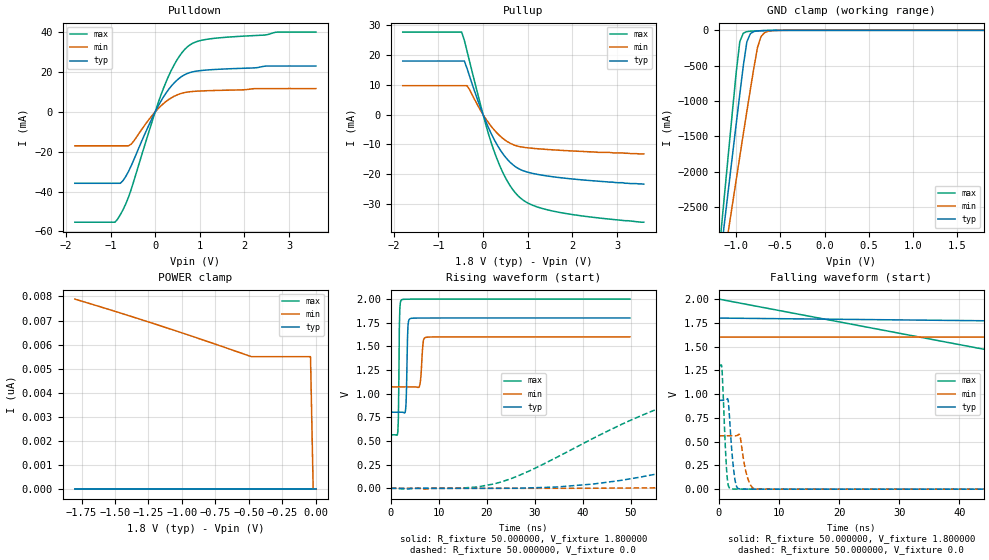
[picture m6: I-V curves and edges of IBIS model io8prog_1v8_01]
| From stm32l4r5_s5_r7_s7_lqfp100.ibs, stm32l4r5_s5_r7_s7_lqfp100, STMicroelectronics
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|   Model io8prog_1v8_01
[Model]  io8prog_1v8_01
Model_type I/O
Polarity   Non-Inverting
Enable   Active-Low
Vinl =   0.540000V
Vinh =   1.260000V
Vmeas =  0.900000V
Cref =   100.000000nF
Rref =   1.000000k
Vref =   1.800000V
C_comp   2.197300pF   2.162700pF   2.264100pF
[Temperature Range]   25.000000   0.125000k   -40.000000
[Pullup Reference]   1.800000V   1.600000V   2.000000V
[Pulldown Reference]   0.0V   0.0V   0.0V
[POWER Clamp Reference]   1.800000V   1.600000V   2.000000V
[GND Clamp Reference]   0.0V   0.0V   0.0V
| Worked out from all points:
|   slope of the pulldown table from 0 to 0.27 V, typ, clamps not added: 26.2 ohm
|   slope of the pullup table from 0 to 0.27 V, typ, clamps not added: 30.1 ohm
|   GND clamp passes 1 mA (typ) near -0.58 V on its own axis
|   rising waveform, R_fixture 50.000000, V_fixture 1.800000: 20-80 % time 248ps typ, 394ps min, 184ps max; typ from 0.804 V to 1.8 V
|   rising waveform, R_fixture 50.000000, V_fixture 0.0: 20-80 % time 65.2ns typ, 116ns min, 36.2ns max; typ from 0 V to 0.934 V
|   falling waveform, R_fixture 50.000000, V_fixture 1.800000: 20-80 % time 75.8ns typ, 121ns min, 63.2ns max; typ from 1.8 V to 0.804 V
|   falling waveform, R_fixture 50.000000, V_fixture 0.0: 20-80 % time 711ps typ, 1.02ns min, 545ps max; typ from 0.934 V to 0 V
[Pulldown]
|Voltage   I(typ)   I(min)   I(max)
-1.8V     -35.82mA   -17.03mA   -55.34mA
-900mV    -35.82mA   -17.03mA   -55.34mA
-840mV    -35.82mA   -17.03mA   -53.76mA
-720mV    -34.49mA   -17.03mA   -49.08mA
-540mV    -27.18mA   -16.22mA   -39.07mA
-60mV     -2.756mA   -1.584mA   -4.227mA
240mV     9.353mA    5.171mA    14.85mA
480mV     15.75mA    8.427mA    25.77mA
720mV     19.29mA    9.947mA    32.62mA
960mV     20.57mA    10.43mA    35.5mA
1.32V     21.27mA    10.74mA    36.91mA
3.6V      23.03mA    11.73mA    40.05mA
[Pullup]
|Voltage   I(typ)   I(min)   I(max)
-1.8V     18.05mA    9.741mA    27.78mA
-480mV    18.05mA    9.741mA    27.78mA
-420mV    18.05mA    9.741mA    25.03mA
-360mV    15.57mA    9.741mA    21.38mA
60mV      -2.268mA   -1.401mA   -3.341mA
240mV     -8.143mA   -5.004mA   -12mA
360mV     -11.31mA   -6.914mA   -16.72mA
540mV     -15mA      -9.056mA   -22.31mA
840mV     -18.52mA   -10.83mA   -28.11mA
1.14V     -19.87mA   -11.38mA   -30.67mA
1.68V     -21.13mA   -11.96mA   -32.81mA
3.6V      -23.4mA    -13.2mA    -36.2mA
[GND_clamp]
|Voltage   I(typ)   I(min)   I(max)
-1.8V     -9.861A    -8.8A      -9.626A
-1.16V    -3.004A    -3.417A    -2.68A
-1.12V    -2.579A    -3.088A    -2.15A
-1.08V    -2.155A    -2.76A     -1.623A
-1V       -1.315A    -2.108A    -586.3mA
-960mV    -900.6mA   -1.784A    -158.3mA
-920mV    -496.8mA   -1.462A    -39.39mA
-880mV    -160.5mA   -1.144A    -17.82mA
-840mV    -45.92mA   -830.3mA   -12.52mA
-760mV    -8.262mA   -243mA     -7.547mA
-680mV    -3.389mA   -33.05mA   -3.833mA
1.8V      0A         0A         0A
[POWER_clamp]
|Voltage   I(typ)   I(min)   I(max)
-1.8V     0A         7.891nA    0A
-1.14V    0A         6.744nA    0A
-480mV    0A         5.5nA      0A
-40mV     0A         5.5nA      0A
-20mV     0A         0A         0A
0V        0A         0A         0A
[Ramp]
| variable   typ   min   max
dV/dt_r  0.56066/65.10411n   0.33689/0.11591u   0.77868/36.15625n
dV/dt_f  0.59736/66.12115n   0.31662/0.11582u   0.86072/35.01231n
R_load = 50.000000
[Rising Waveform]
R_fixture= 50.000000
V_fixture= 1.800000
V_fixture_min= 1.600000
V_fixture_max= 2.000000
|time   V(typ)   V(min)   V(max)
0s        804.4mV    1.072V     565.5mV
1.502ns   804.4mV    1.072V     605.1mV
1.902ns   804.4mV    1.072V     1.897V
2.302ns   804.2mV    1.072V     1.993V
3.103ns   828.2mV    1.072V     1.998V
3.604ns   1.718V     1.072V     1.999V
4.104ns   1.794V     1.072V     1.999V
6.006ns   1.8V       1.08V      2V
7.407ns   1.8V       1.596V     2V
49.85ns   1.8V       1.6V       2V
[Rising Waveform]
R_fixture= 50.000000
V_fixture= 0.0
V_fixture_min= 0.0
V_fixture_max= 0.0
|time   V(typ)   V(min)   V(max)
0s        1.798uV    1.954uV    2.437uV
21.62ns   330uV      -33.39uV   47.64mV
42.04ns   44.71mV    937uV      524.5mV
64.86ns   250.4mV    13.63mV    994.4mV
81.68ns   427.8mV    39.23mV    1.169V
102.1ns   611.1mV    97.11mV    1.25V
127.3ns   762.8mV    186.7mV    1.28V
156.2ns   853.2mV    286mV      1.293V
260.7ns   929.8mV    499.2mV    1.298V
598.2ns   934.4mV    561.5mV    1.298V
[Falling Waveform]
R_fixture= 50.000000
V_fixture= 1.800000
V_fixture_min= 1.600000
V_fixture_max= 2.000000
|time   V(typ)   V(min)   V(max)
0s        1.8V       1.6V       2V
50.05ns   1.768V     1.6V       1.4V
100.1ns   1.333V     1.566V     660.4mV
150.2ns   966.2mV    1.432V     586.8mV
200.2ns   866.1mV    1.275V     571.3mV
250.2ns   829.7mV    1.173V     567mV
300.3ns   815.2mV    1.131V     566.1mV
400.4ns   806.4mV    1.091V     565.5mV
550.6ns   804.6mV    1.076V     565.5mV
4.955us   804.4mV    1.072V     565.5mV
[Falling Waveform]
R_fixture= 50.000000
V_fixture= 0.0
V_fixture_min= 0.0
V_fixture_max= 0.0
|time   V(typ)   V(min)   V(max)
0s        934.4mV    561.5mV    1.298V
500.5ps   934.7mV    561.5mV    1.303V
1.401ns   946mV      561.6mV    139.5mV
1.602ns   928.7mV    561.7mV    40.99mV
2.002ns   569mV      561.8mV    5.392mV
2.703ns   104mV      561.4mV    1.238mV
3.403ns   4.316mV    577.3mV    759.5uV
4.805ns   557.2uV    119.3mV    433.8uV
6.006ns   271.8uV    3.014mV    295.9uV
49.85ns   1.798uV    1.954uV    2.437uV
